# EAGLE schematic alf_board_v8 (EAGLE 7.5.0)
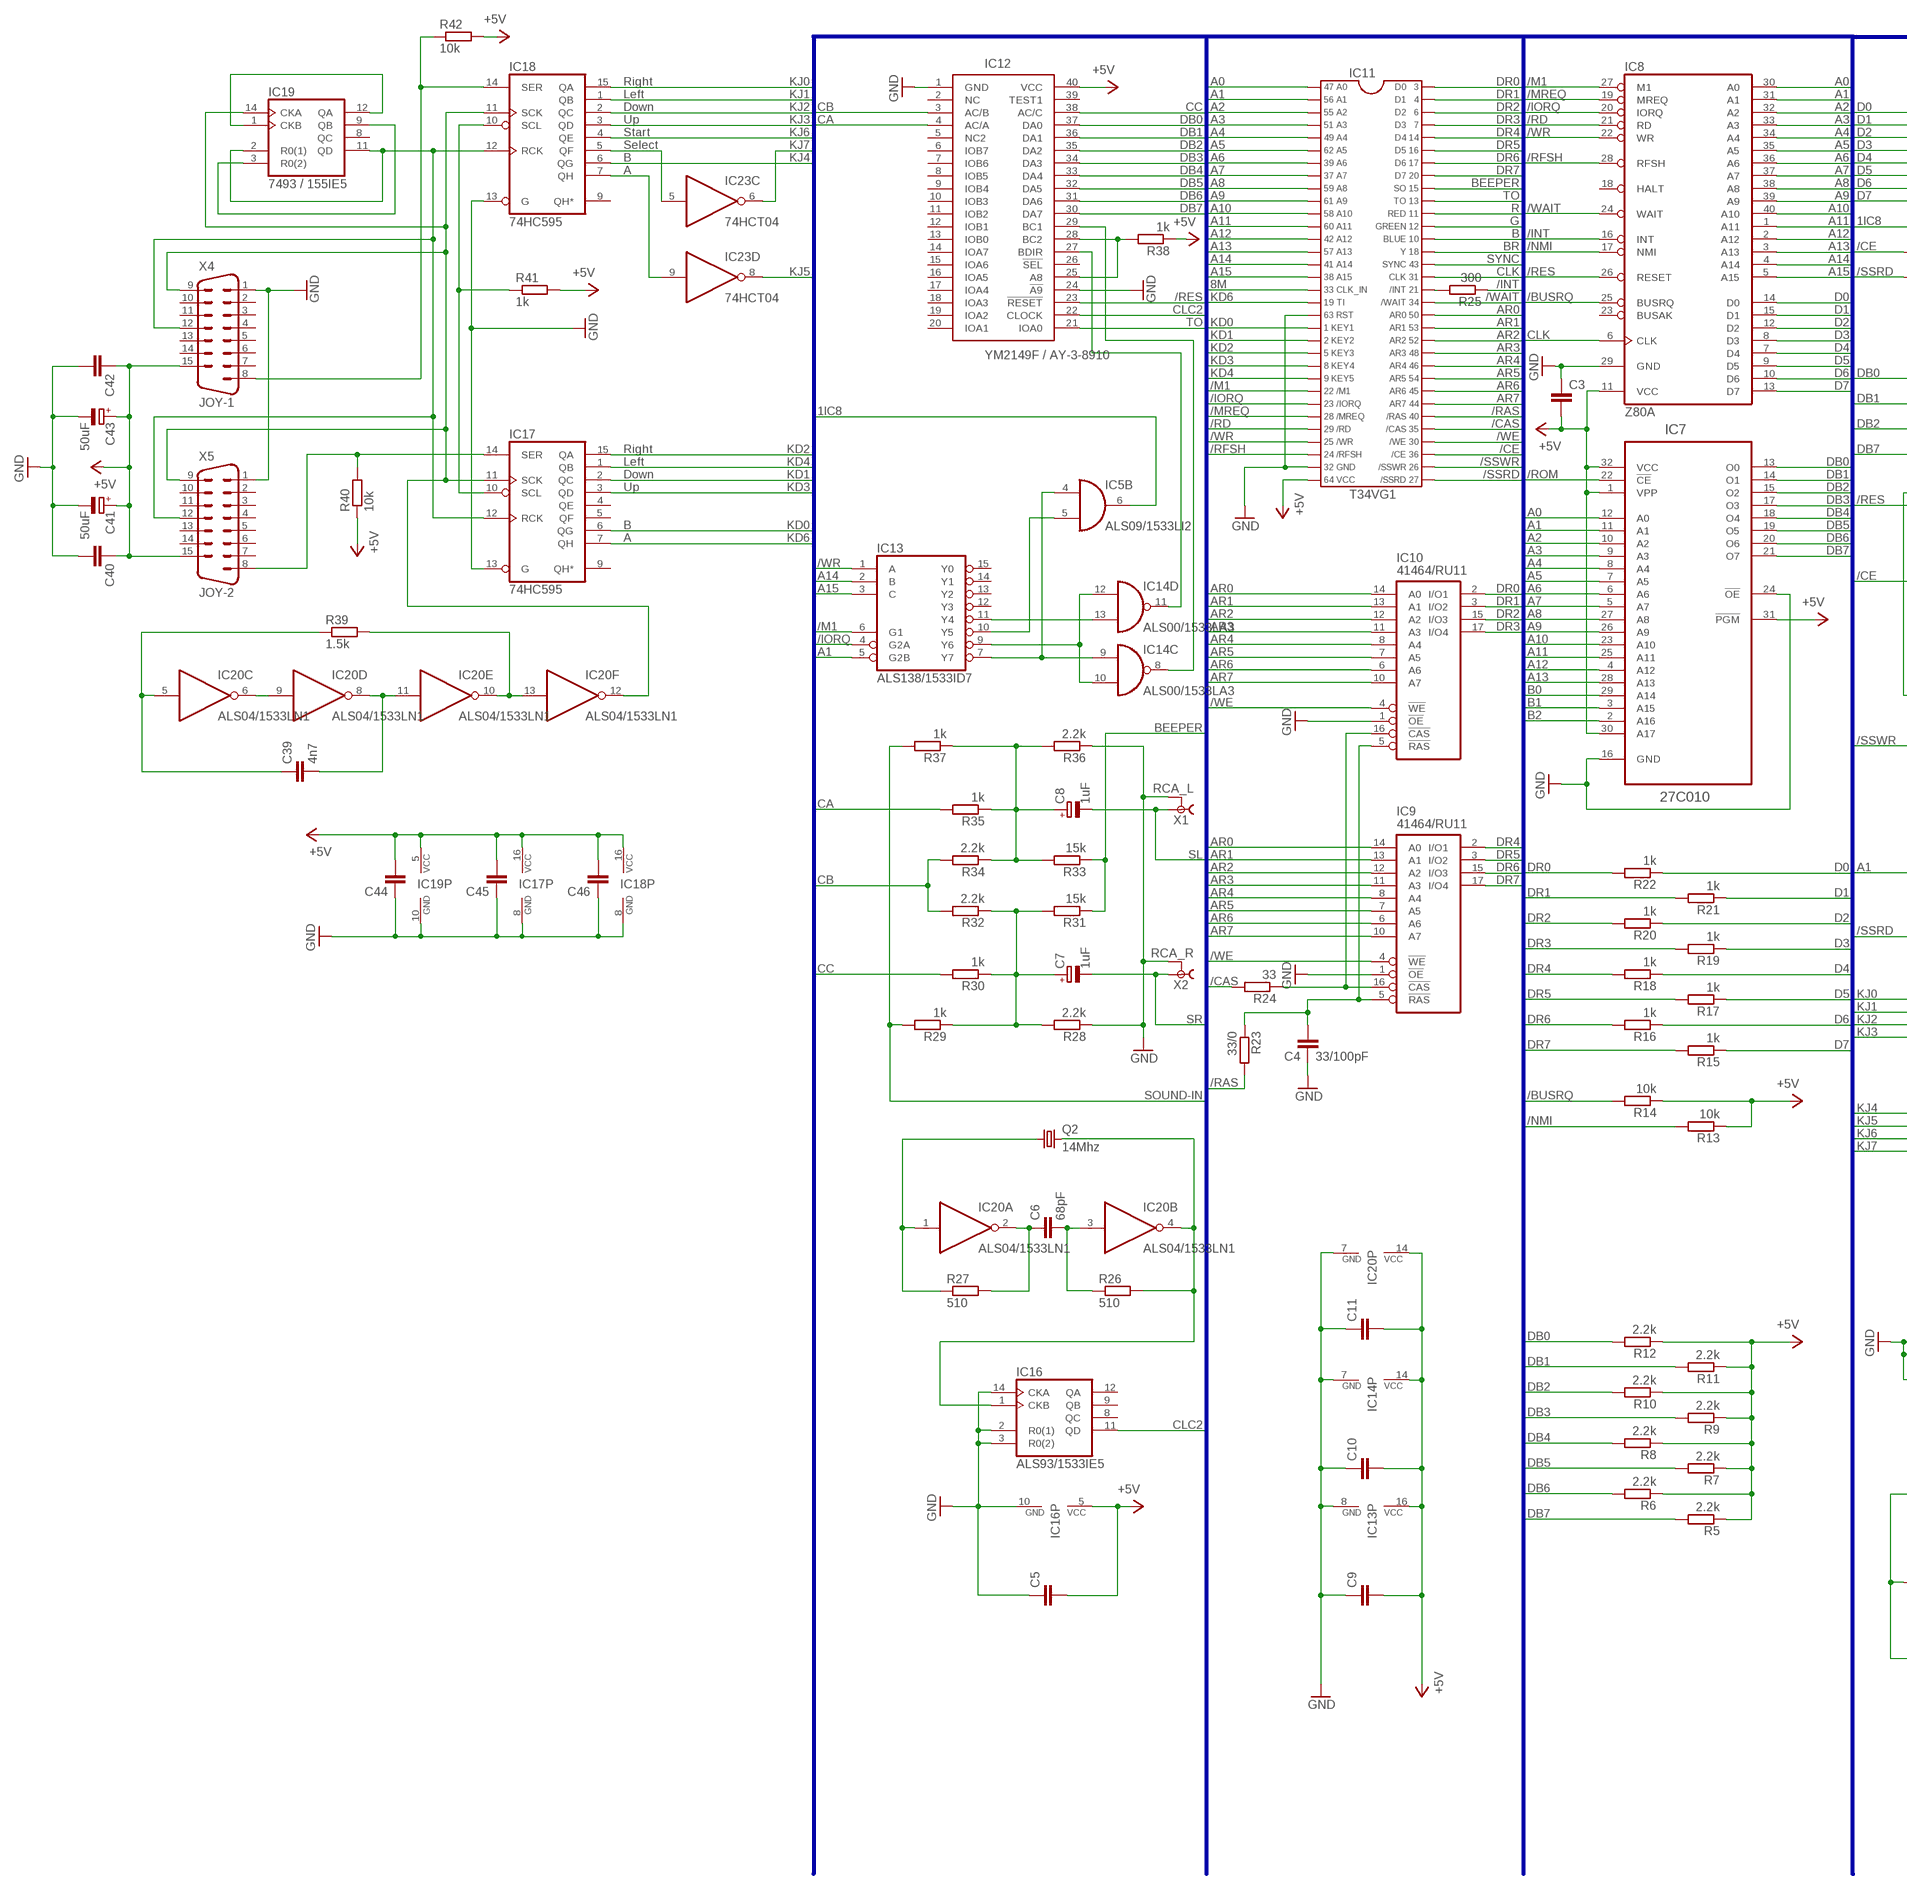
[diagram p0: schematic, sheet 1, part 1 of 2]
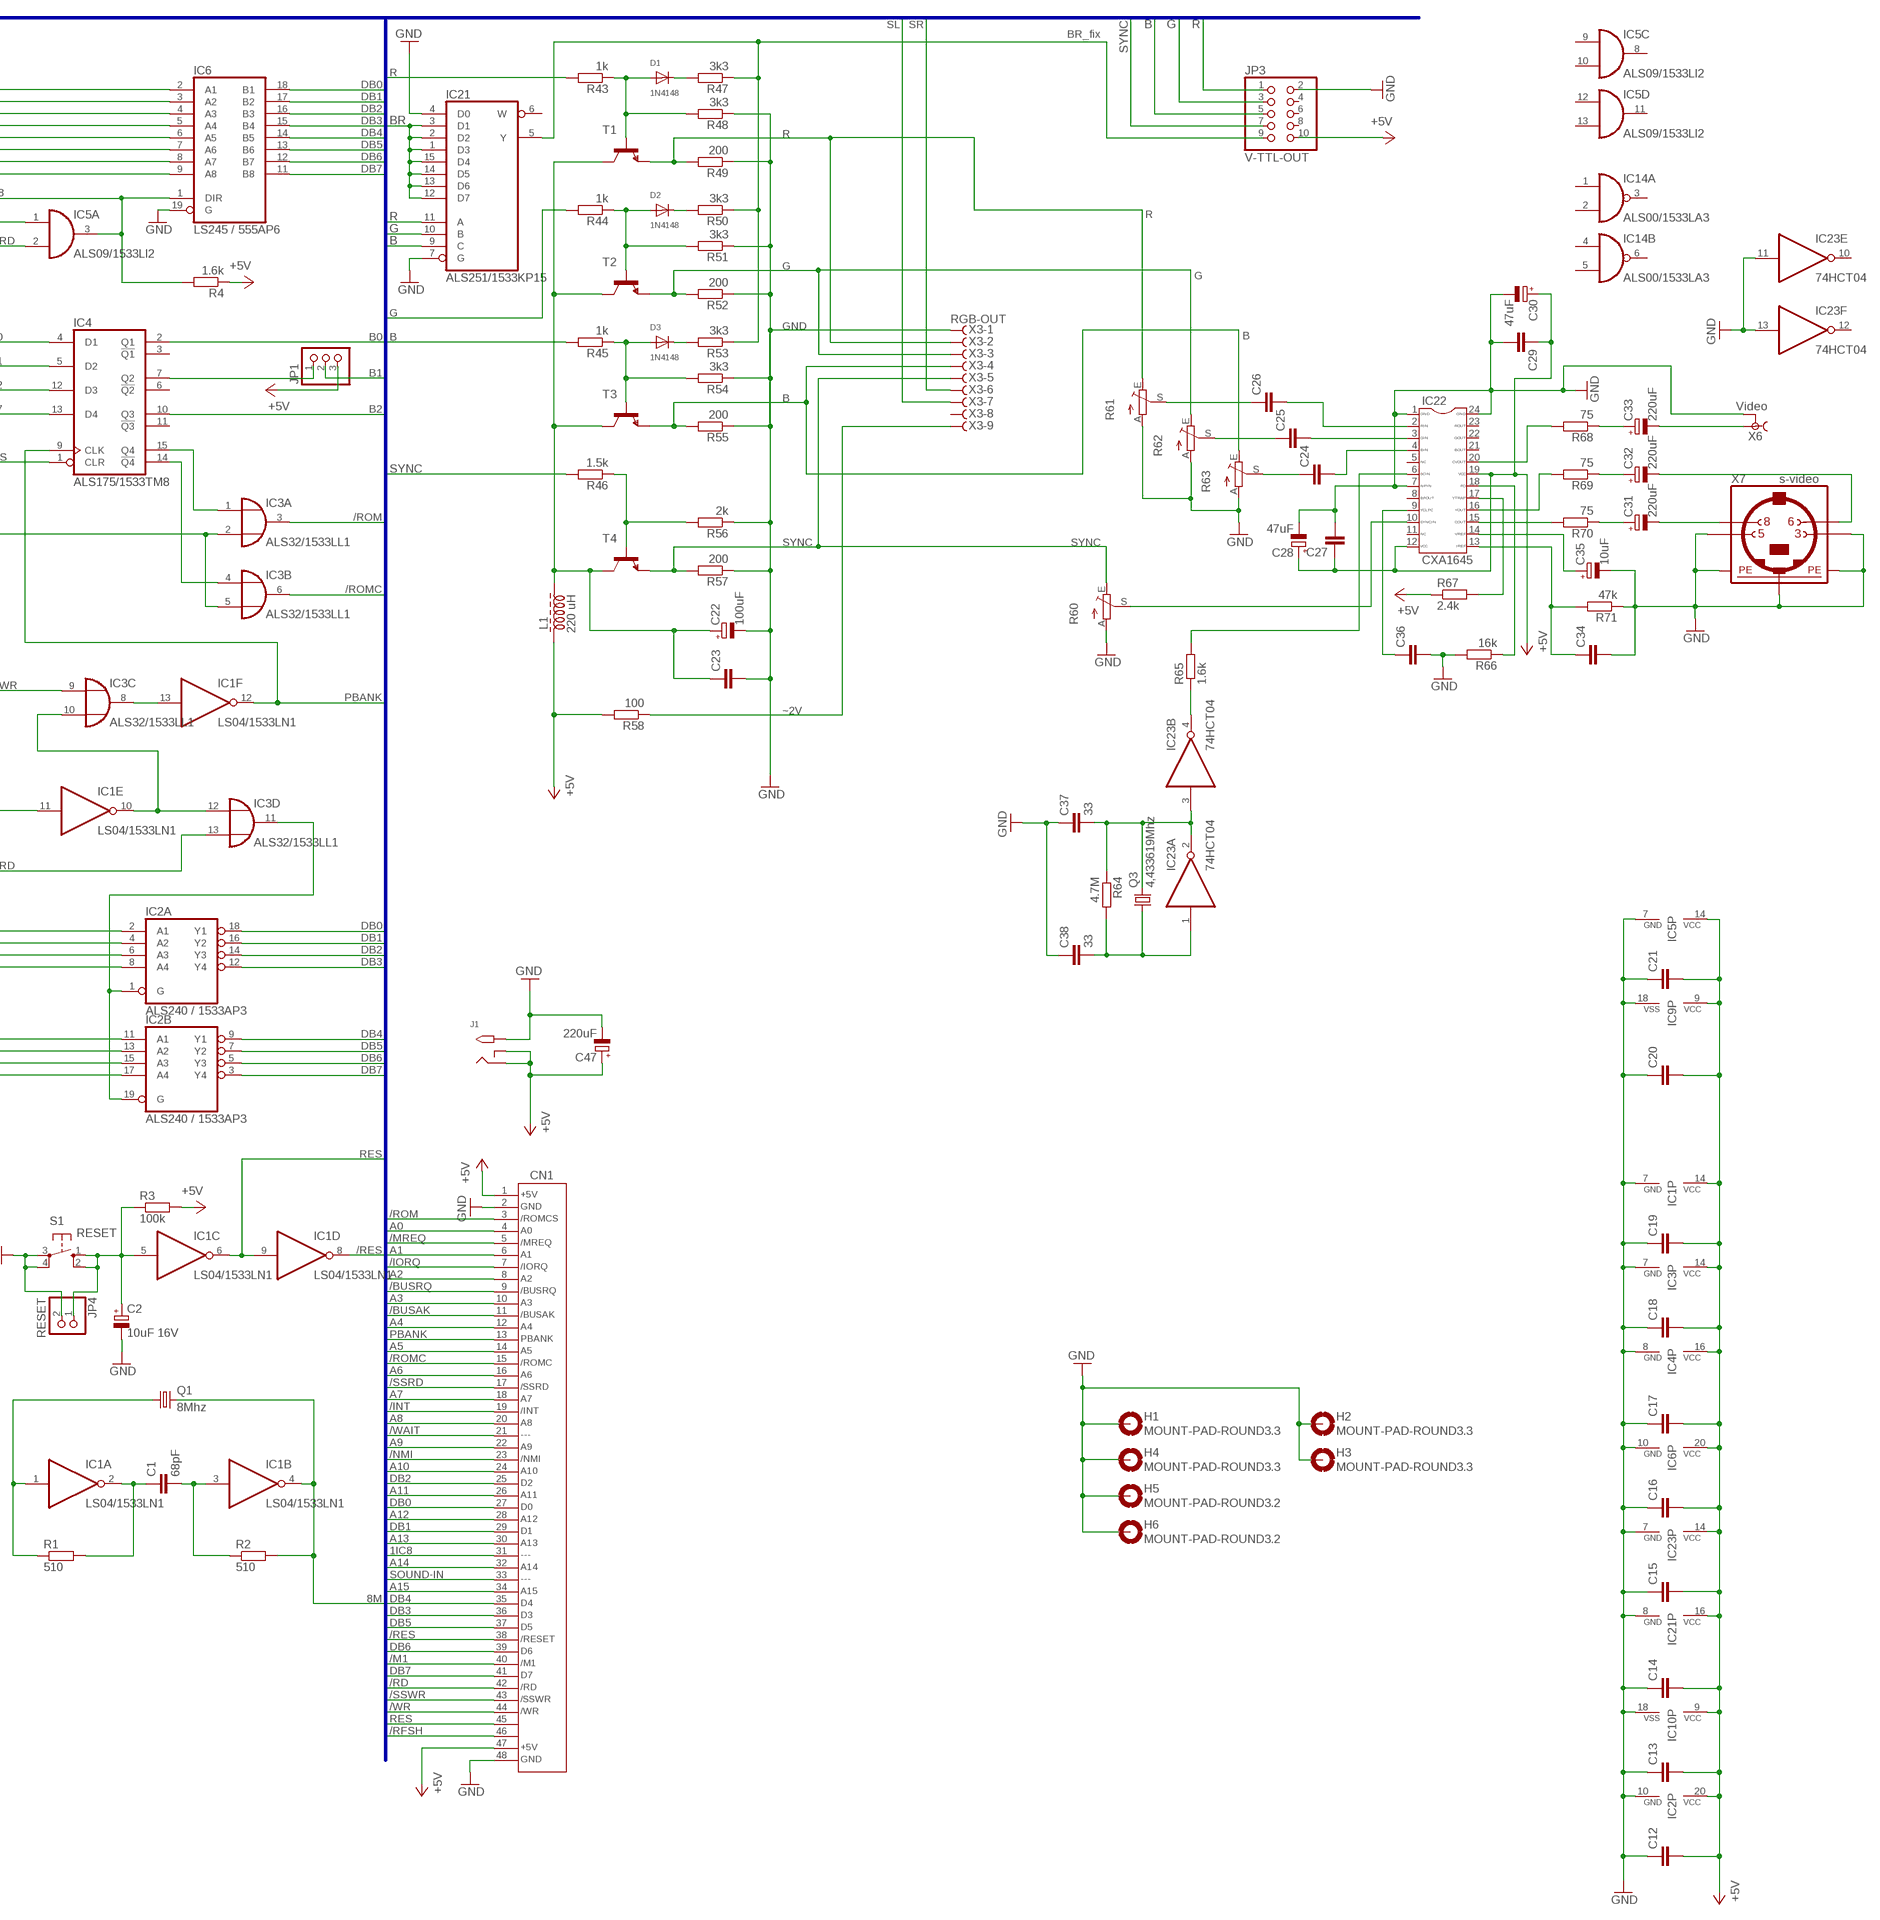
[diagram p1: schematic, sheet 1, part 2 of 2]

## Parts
C1  68pF  C-EUC0805  [C0805]
C2  10uF 16V  CPOL-EUSMCA  [SMC_A]
C3  C-EUC0805  [C0805]
C4  33/100pF  C-EUC0805  [C0805]
C5  C-EUC0805  [C0805]
C6  68pF  C-EUC0805  [C0805]
C7  1uF  CPOL-EUSMCA  [SMC_A]
C8  1uF  CPOL-EUSMCA  [SMC_A]
C9  C-EUC0805  [C0805]
C10  C-EUC0805  [C0805]
C11  C-EUC0805  [C0805]
C12  C-EUC0805  [C0805]
C13  C-EUC0805  [C0805]
C14  C-EUC0805  [C0805]
C15  C-EUC0805  [C0805]
C16  C-EUC0805  [C0805]
C17  C-EUC0805  [C0805]
C18  C-EUC0805  [C0805]
C19  C-EUC0805  [C0805]
C20  C-EUC0805  [C0805]
C21  C-EUC0805  [C0805]
C22  100uF  CPOL-EUSMCB  [SMC_B]
C23  C-EUC0805  [C0805]
C24  C-EUC0805  [C0805]
C25  C-EUC0805  [C0805]
C26  C-EUC0805  [C0805]
C27  C-EUC0805  [C0805]
C28  47uF  CPOL-EUSMCB  [SMC_B]
C29  C-EUC0805  [C0805]
C30  47uF  CPOL-EUSMCB  [SMC_B]
C31  220uF  CPOL-EUSMCD  [SMC_D]
C32  220uF  CPOL-EUSMCD  [SMC_D]
C33  220uF  CPOL-EUSMCD  [SMC_D]
C34  C-EUC0805  [C0805]
C35  10uF  CPOL-EUSMCA  [SMC_A]
C36  C-EUC0805  [C0805]
C37  33  C-EUC0805  [C0805]
C38  33  C-EUC0805  [C0805]
C39  4n7  C-EUC0805  [C0805]
C40  C-EUC0805  [C0805]
C41  50uF  CPOL-EUSMCB  [SMC_B]
C42  C-EUC0805  [C0805]
C43  50uF  CPOL-EUSMCB  [SMC_B]
C44  C-EUC0805  [C0805]
C45  C-EUC0805  [C0805]
C46  C-EUC0805  [C0805]
C47  220uF  CPOL-EUSMCD  [SMC_D]
CN1  СНП15-48  [СНП15-48]
D1  1N4148  DIODEDO-1N4148  [DO-1N4148]
D2  1N4148  DIODEDO-1N4148  [DO-1N4148]
D3  1N4148  DIODEDO-1N4148  [DO-1N4148]
H1  MOUNT-PAD-ROUND3.3  [3,3-PAD]
H2  MOUNT-PAD-ROUND3.3  [3,3-PAD]
H3  MOUNT-PAD-ROUND3.3  [3,3-PAD]
H4  MOUNT-PAD-ROUND3.3  [3,3-PAD]
H5  MOUNT-PAD-ROUND3.2  [3,2-PAD]
H6  MOUNT-PAD-ROUND3.2  [3,2-PAD]
IC1  LS04/1533LN1  74LS04N  [DIL14]
IC2  ALS240 / 1533AP3  74LS240N  [DIL20]
IC3  ALS32/1533LL1  74LS32N  [DIL14]
IC4  ALS175/1533TM8  74LS175N  [DIL16]
IC5  ALS09/1533LI2  74LS09N  [DIL14]
IC6  LS245 / 555AP6  74LS245N  [DIL20]
IC7  27C010  AT27C020-90PU  [DIP254P1524X482-32P]
IC8  Z80A  Z80CPU  [DIL40]
IC9  41464/RU11  41464  [DIL18]
IC10  41464/RU11  41464  [DIL18]
IC11  T34VG1  Т34ВГ1  [TQFP64]
IC12  YM2149F / AY-3-8910  YM2149F  [DIL40]
IC13  ALS138/1533ID7  74LS138N  [DIL16]
IC14  ALS00/1533LA3  74LS00N  [DIL14]
IC16  ALS93/1533IE5  74LS93N  [DIL14]
IC17  74HC595  74HC595N  [DIL16]
IC18  74HC595  74HC595N  [DIL16]
IC19  7493 / 155IE5  74LS93N  [DIL14]
IC20  ALS04/1533LN1  74LS04N  [DIL14]
IC21  ALS251/1533KP15  74LS251N  [DIL16]
IC22  CXA1645  [SOP24]
IC23  74HCT04  74HCT04N  [DIL14]
J1  2.1MMJACKTHM  [PJ-102A]
JP1  PINHD-1X3  [1X03]
JP3  V-TTL-OUT  PINHD-2X5  [2X05]
JP4  RESET  PINHD-1X2  [1X02]
L1  220 uH  Z27/24CW  [Z27/24]
Q1  8Mhz  CRYSTALHC49S  [HC49/S]
Q2  14Mhz  CRYSTALHC49S  [HC49/S]
Q3  4,433619Mhz  CRYSTALHC49S  [HC49/S]
R1  510  R-EU_R0805  [R0805]
R2  510  R-EU_R0805  [R0805]
R3  100k  R-EU_R0805  [R0805]
R4  1.6k  R-EU_R0805  [R0805]
R5  2.2k  R-EU_R0805  [R0805]
R6  2.2k  R-EU_R0805  [R0805]
R7  2.2k  R-EU_R0805  [R0805]
R8  2.2k  R-EU_R0805  [R0805]
R9  2.2k  R-EU_R0805  [R0805]
R10  2.2k  R-EU_R0805  [R0805]
R11  2.2k  R-EU_R0805  [R0805]
R12  2.2k  R-EU_R0805  [R0805]
R13  10k  R-EU_R0805  [R0805]
R14  10k  R-EU_R0805  [R0805]
R15  1k  R-EU_R0805  [R0805]
R16  1k  R-EU_R0805  [R0805]
R17  1k  R-EU_R0805  [R0805]
R18  1k  R-EU_R0805  [R0805]
R19  1k  R-EU_R0805  [R0805]
R20  1k  R-EU_R0805  [R0805]
R21  1k  R-EU_R0805  [R0805]
R22  1k  R-EU_R0805  [R0805]
R23  33/0  R-EU_R0805  [R0805]
R24  33  R-EU_R0805  [R0805]
R25  300  R-EU_R0805  [R0805]
R26  510  R-EU_R0805  [R0805]
R27  510  R-EU_R0805  [R0805]
R28  2.2k  R-EU_R0805  [R0805]
R29  1k  R-EU_R0805  [R0805]
R30  1k  R-EU_R0805  [R0805]
R31  15k  R-EU_R0805  [R0805]
R32  2.2k  R-EU_R0805  [R0805]
R33  15k  R-EU_R0805  [R0805]
R34  2.2k  R-EU_R0805  [R0805]
R35  1k  R-EU_R0805  [R0805]
R36  2.2k  R-EU_R0805  [R0805]
R37  1k  R-EU_R0805  [R0805]
R38  1k  R-EU_R0805  [R0805]
R39  1.5k  R-EU_R0805  [R0805]
R40  10k  R-EU_R0805  [R0805]
R41  1k  R-EU_R0805  [R0805]
R42  10k  R-EU_R0805  [R0805]
R43  1k  R-EU_R0805  [R0805]
R44  1k  R-EU_R0805  [R0805]
R45  1k  R-EU_R0805  [R0805]
R46  1.5k  R-EU_R0805  [R0805]
R47  3k3  R-EU_R0805  [R0805]
R48  3k3  R-EU_R0805  [R0805]
R49  200  R-EU_R0805  [R0805]
R50  3k3  R-EU_R0805  [R0805]
R51  3k3  R-EU_R0805  [R0805]
R52  200  R-EU_R0805  [R0805]
R53  3k3  R-EU_R0805  [R0805]
R54  3k3  R-EU_R0805  [R0805]
R55  200  R-EU_R0805  [R0805]
R56  2k  R-EU_R0805  [R0805]
R57  200  R-EU_R0805  [R0805]
R58  100  R-EU_R0805  [R0805]
R60  TRIM_EU-CA6V  [CA6V]
R61  TRIM_EU-CA6V  [CA6V]
R62  TRIM_EU-CA6V  [CA6V]
R63  TRIM_EU-CA6V  [CA6V]
R64  4.7M  R-EU_R0805  [R0805]
R65  1.6k  R-EU_R0805  [R0805]
R66  16k  R-EU_R0805  [R0805]
R67  2.4k  R-EU_R0805  [R0805]
R68  75  R-EU_R0805  [R0805]
R69  75  R-EU_R0805  [R0805]
R70  75  R-EU_R0805  [R0805]
R71  47k  R-EU_R0805  [R0805]
S1  RESET  10-XX  [B3F-10XX]
T1  BC549-NPN-TO92-CBE  [TO92-CBE]
T2  BC549-NPN-TO92-CBE  [TO92-CBE]
T3  BC549-NPN-TO92-CBE  [TO92-CBE]
T4  BC549-NPN-TO92-CBE  [TO92-CBE]
X1  RCA_L  TOBU3  [TOBU3]
X2  RCA_R  TOBU3  [TOBU3]
X3  RGB-OUT  D-SUB9-H5M09RA  [H5M09RA]
X4  JOY-1  M15HP  [M15HP]
X5  JOY-2  M15HP  [M15HP]
X6  Video  TOBU3  [TOBU3]
X7  s-video  MINI_DIN_4  [M_DIN4]

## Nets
1IC8: CN1.31 IC5.3(A:O) IC5.6(B:O) IC6.1(DIR) R4.2
8M: IC1.4(B:O) IC11.33 Q1.2 R2.2
+5V: C3.2 C5.2 C9.2 C10.2 C11.2 C12.2 C13.2 C14.2 C15.2 C16.2 C17.2 C18.2 C19.2 C20.2 C21.2 C27.1 C28.+ C29.1 C30.+ C40.1 C41.+ C42.1 C43.+ C44.2 C45.2 C46.2 C47.+ CN1.1 CN1.47 IC1.14(P:VCC) IC2.20(P:VCC) IC3.14(P:VCC) IC4.16(VCC) IC5.14(P:VCC) IC6.20(VCC) IC7.1(VPP) IC7.30(A17) IC7.31(!PGM) IC7.32(VCC) IC8.11(VCC) IC9.9(VCC) IC10.9(VCC) IC11.64 IC12.40(VCC) IC13.16(VCC) IC14.14(P:VCC) IC16.5(VCC) IC17.16(VCC) IC18.16(VCC) IC19.5(VCC) IC20.14(P:VCC) IC21.16(VCC) IC22.12 IC22.19 IC23.14(P:VCC) J1.RING J1.RING_SW JP1.3 JP3.10 L1.1 R3.2 R4.1 R5.1 R6.1 R7.1 R8.1 R9.1 R10.1 R11.1 R12.1 R13.1 R14.1 R38.1 R40.1 R41.2 R42.2 R58.2 R67.1 X4.15 X5.15
/BUSAK: CN1.11
/BUSRQ: CN1.9 IC8.25(BUSRQ) R14.2
/CAS: IC11.35 R24.2
/CE: IC3.2(A:I1) IC3.5(B:I1) IC5.1(A:I0) IC11.36
/INT: CN1.19 IC8.16(INT) R25.1
/IORQ: CN1.7 IC8.20(IORQ) IC11.23 IC13.4(G2A)
/M1: CN1.40 IC8.27(M1) IC11.22 IC13.6(G1)
/MREQ: CN1.5 IC8.19(MREQ) IC11.28
/NMI: CN1.23 IC8.17(NMI) R13.2
/RAS: IC11.40 R23.2
/RD: CN1.42 IC8.21(RD) IC11.29
/RES: CN1.38 IC1.8(D:O) IC4.1(CLR) IC8.26(RESET) IC12.23(!RESET)
/RFSH: CN1.46 IC8.28(RFSH) IC11.24
/ROM: CN1.3 IC3.3(A:O) IC7.22(!CE)
/ROMC: CN1.15 IC3.6(B:O)
/SSRD: CN1.17 IC3.13(D:I1) IC5.2(A:I1) IC11.27
/SSWR: CN1.43 IC3.9(C:I0) IC11.26
/WAIT: CN1.21 IC8.24(WAIT) IC11.34
/WE: IC9.4(!WE) IC10.4(!WE) IC11.30
/WR: CN1.44 IC8.22(WR) IC11.25 IC13.1(A)
A0: CN1.4 IC7.12(A0) IC8.30(A0) IC11.47
A1: CN1.6 IC1.11(E:I) IC7.11(A1) IC8.31(A1) IC11.56 IC13.5(G2B)
A2: CN1.8 IC7.10(A2) IC8.32(A2) IC11.55
A3: CN1.10 IC7.9(A3) IC8.33(A3) IC11.51
A4: CN1.12 IC7.8(A4) IC8.34(A4) IC11.49
A5: CN1.14 IC7.7(A5) IC8.35(A5) IC11.62
A6: CN1.16 IC7.6(A6) IC8.36(A6) IC11.39
A7: CN1.18 IC7.5(A7) IC8.37(A7) IC11.37
A8: CN1.20 IC7.27(A8) IC8.38(A8) IC11.59
A9: CN1.22 IC7.26(A9) IC8.39(A9) IC11.61
A10: CN1.24 IC7.23(A10) IC8.40(A10) IC11.58
A11: CN1.26 IC7.25(A11) IC8.1(A11) IC11.60
A12: CN1.28 IC7.4(A12) IC8.2(A12) IC11.42
A13: CN1.30 IC7.28(A13) IC8.3(A13) IC11.57
A14: CN1.32 IC8.4(A14) IC11.41 IC13.2(B)
A15: CN1.34 IC8.5(A15) IC11.38 IC13.3(C)
AR0: IC9.14(A0) IC10.14(A0) IC11.50
AR1: IC9.13(A1) IC10.13(A1) IC11.53
AR2: IC9.12(A2) IC10.12(A2) IC11.52
AR3: IC9.11(A3) IC10.11(A3) IC11.48
AR4: IC9.8(A4) IC10.8(A4) IC11.46
AR5: IC9.7(A5) IC10.7(A5) IC11.54
AR6: IC9.6(A6) IC10.6(A6) IC11.45
AR7: IC9.10(A7) IC10.10(A7) IC11.44
B: IC11.10 IC21.9(C) JP3.5 R45.2
B0: IC4.2(Q1) IC7.29(A14)
B1: IC7.3(A15) JP1.2
B2: IC4.10(Q3) IC7.2(A16)
BEEPER: IC11.15 R31.1 R33.1
BR: IC11.18 IC21.1(D3) IC21.2(D2) IC21.3(D1) IC21.12(D7) IC21.13(D6) IC21.14(D5) IC21.15(D4)
CA: IC12.4(AC/A) R35.2
CB: IC12.3(AC/B) R32.2 R34.2
CC: IC12.38(AC/C) R30.2
CLC2: IC12.22(CLOCK) IC16.11(QD)
CLK: IC8.6(CLK) IC11.31
D0: IC6.2(A1) IC8.14(D0) R22.1
D1: IC6.3(A2) IC8.15(D1) R21.1
D2: IC6.4(A3) IC8.12(D2) R20.1
D3: IC6.5(A4) IC8.8(D3) R19.1
D4: IC6.6(A5) IC8.7(D4) R18.1
D5: IC6.7(A6) IC8.9(D5) R17.1
D6: IC6.8(A7) IC8.10(D6) R16.1
D7: IC6.9(A8) IC8.13(D7) R15.1
DB0: CN1.27 IC2.18(A:Y1) IC4.4(D1) IC6.18(B1) IC7.13(O0) IC12.37(DA0) R12.2
DB1: CN1.29 IC2.16(A:Y2) IC4.5(D2) IC6.17(B2) IC7.14(O1) IC12.36(DA1) R11.2
DB2: CN1.25 IC2.14(A:Y3) IC4.12(D3) IC6.16(B3) IC7.15(O2) IC12.35(DA2) R10.2
DB3: CN1.36 IC2.12(A:Y4) IC6.15(B4) IC7.17(O3) IC12.34(DA3) R9.2
DB4: CN1.35 IC2.9(B:Y1) IC6.14(B5) IC7.18(O4) IC12.33(DA4) R8.2
DB5: CN1.37 IC2.7(B:Y2) IC6.13(B6) IC7.19(O5) IC12.32(DA5) R7.2
DB6: CN1.39 IC2.5(B:Y3) IC6.12(B7) IC7.20(O6) IC12.31(DA6) R6.2
DB7: CN1.41 IC2.3(B:Y4) IC4.13(D4) IC6.11(B8) IC7.21(O7) IC12.30(DA7) R5.2
DR0: IC10.2(I/O1) IC11.3 R22.2
DR1: IC10.3(I/O2) IC11.4 R21.2
DR2: IC10.15(I/O3) IC11.6 R20.2
DR3: IC10.17(I/O4) IC11.7 R19.2
DR4: IC9.2(I/O1) IC11.14 R18.2
DR5: IC9.3(I/O2) IC11.16 R17.2
DR6: IC9.15(I/O3) IC11.17 R16.2
DR7: IC9.17(I/O4) IC11.20 R15.2
G: IC11.12 IC21.10(B) JP3.3 R44.2
GND: C2.- C3.1 C4.1 C5.1 C9.1 C10.1 C11.1 C12.1 C13.1 C14.1 C15.1 C16.1 C17.1 C18.1 C19.1 C20.1 C21.1 C22.- C23.2 C27.2 C28.- C29.2 C30.- C34.2 C35.- C36.2 C37.1 C38.1 C40.2 C41.- C42.2 C43.- C44.1 C45.1 C46.1 C47.- CN1.2 CN1.48 H1.B3,3(MOUNT) H2.B3,3(MOUNT) H3.B3,3(MOUNT) H4.B3,3(MOUNT) H5.B3,2(MOUNT) H6.B3,2(MOUNT) IC1.7(P:GND) IC2.10(P:GND) IC3.7(P:GND) IC4.8(GND) IC5.7(P:GND) IC6.10(GND) IC6.19(G) IC7.16(GND) IC7.24(!OE) IC8.29(GND) IC9.1(!OE) IC9.18(VSS) IC10.1(!OE) IC10.18(VSS) IC11.32 IC11.63 IC12.1(GND) IC12.24(!A9) IC13.8(GND) IC14.7(P:GND) IC16.2(R0(1)) IC16.3(R0(2)) IC16.10(GND) IC16.14(CKA) IC17.8(GND) IC17.13(G) IC18.8(GND) IC18.13(G) IC19.10(GND) IC20.7(P:GND) IC21.4(D0) IC21.7(G) IC21.8(GND) IC22.1 IC22.7 IC22.24 IC23.7(P:GND) IC23.11(E:I) IC23.13(F:I) J1.TIP JP3.2 JP4.2 R28.1 R36.1 R48.1 R49.1 R51.1 R52.1 R54.1 R55.1 R56.1 R57.1 R60.A R61.A R62.A R63.A R66.2 R71.1 S1.3(P) S1.4(P1) X1.2 X1.2@1 X1.2@2 X2.2 X2.2@1 X2.2@2 X3.1 X4.1 X5.1 X6.2 X6.2@1 X6.2@2 X7.3 X7.5 X7.SH1(PE1) X7.SH2(PE2) X7.SH3(PE3)
KD0: IC11.1 IC17.6(QG)
KD1: IC11.2 IC17.2(QC)
KD2: IC11.5 IC17.15(QA)
KD3: IC11.8 IC17.3(QD)
KD4: IC11.9 IC17.1(QB)
KD6: IC11.19 IC17.7(QH)
KJ0: IC2.2(A:A1) IC18.15(QA)
KJ1: IC2.4(A:A2) IC18.1(QB)
KJ2: IC2.6(A:A3) IC18.2(QC)
KJ3: IC2.8(A:A4) IC18.3(QD)
KJ4: IC2.11(B:A1) IC18.6(QG)
KJ5: IC2.13(B:A2) IC23.8(D:O)
KJ6: IC2.15(B:A3) IC18.4(QE)
KJ7: IC2.17(B:A4) IC23.6(C:O)
N$1: IC23.4(B:O) R65.1
N$2: C1.1 IC1.2(A:O) R1.2
N$3: C1.2 IC1.3(B:I) R2.1
N$4: IC1.1(A:I) Q1.1 R1.1
N$5: IC18.5(QF) IC23.5(C:I)
N$6: IC18.7(QH) IC23.9(D:I)
N$7: IC1.13(F:I) IC3.8(C:O)
N$8: C2.+ IC1.5(C:I) JP4.1 R3.1 S1.1(S) S1.2(S1)
N$9: IC4.7(Q2) JP1.1
N$10: IC1.10(E:O) IC3.10(C:I1) IC3.12(D:I0)
N$11: IC3.4(B:I0) IC4.14(!Q4)
N$12: IC2.1(A:G) IC2.19(B:G) IC3.11(D:O)
N$13: IC3.1(A:I0) IC4.15(Q4)
N$14: IC17.12(RCK) IC18.12(RCK) IC19.2(R0(1)) IC19.11(QD) X4.12 X5.12
N$15: IC11.21 R25.2
N$16: IC12.25(A8) IC12.28(BC2) R38.2
N$17: D1.A R43.1 R48.2 T1.B
N$18: D1.C R47.2
N$19: R49.2 R61.E T1.E X3.2
N$21: D2.A R44.1 R51.2 T2.B
N$22: D2.C R50.2
N$23: R52.2 R62.E T2.E X3.3
N$24: IC22.17 R67.2
N$25: IC12.27(BDIR) IC14.11(D:O)
N$26: IC5.4(B:I0) IC13.7(Y7) IC14.9(C:I0)
N$27: IC13.11(Y4) IC14.13(D:I1)
N$28: IC5.5(B:I1) IC13.10(Y5)
N$29: IC13.9(Y6) IC14.10(C:I1) IC14.12(D:I0)
N$30: IC17.10(SCL) IC18.10(SCL) R41.1
N$31: IC12.29(BC1) IC14.8(C:O)
N$32: C8.+ R33.2 R34.1 R35.1 R36.2 R37.1
N$33: C7.+ R28.2 R29.1 R30.1 R31.2 R32.1
N$34: D3.A R45.1 R54.2 T3.B
N$35: IC17.11(SCK) IC18.11(SCK) IC19.14(CKA) IC20.12(F:O) X4.9 X5.9
N$36: C39.1 IC20.5(C:I) R39.1
N$37: IC16.1(CKB) IC20.4(B:O) Q2.2 R26.2
N$38: IC20.1(A:I) Q2.1 R27.1
N$39: C6.1 IC20.2(A:O) R27.2
N$40: C6.2 IC20.3(B:I) R26.1
N$41: D3.C R53.2
N$42: R55.2 R63.E T3.E X3.4
N$43: R57.2 R60.E T4.E X3.5
N$44: C22.+ C23.1 L1.2 T1.C T2.C T3.C T4.C
N$45: R58.1 X3.9
N$46: IC17.14(SER) R40.2 X5.8
N$47: IC19.3(R0(2)) IC19.9(QB)
N$48: IC18.14(SER) R42.1 X4.8
N$49: IC19.1(CKB) IC19.12(QA)
N$50: C39.2 IC20.8(D:O) IC20.11(E:I)
N$51: IC20.10(E:O) IC20.13(F:I) R39.2
N$52: C26.1 R61.S
N$53: IC20.6(C:O) IC20.9(D:I)
N$54: C25.1 R62.S
N$55: C24.1 R63.S
N$56: C25.2 IC22.3
N$57: C26.2 IC22.2
N$58: C24.2 IC22.4
N$59: C38.2 IC23.1(A:I) Q3.1 R64.2
N$60: C37.2 IC23.2(A:O) IC23.3(B:I) Q3.2 R64.1
N$61: IC22.10 R60.S
N$62: IC21.5(Y) JP3.9 R47.1 R50.1 R53.1
N$63: IC22.6 R65.2
N$64: IC22.20 R68.2
N$65: C36.1 IC22.9
N$66: IC22.18 R66.1
N$67: IC22.16 R69.2
N$68: IC22.15 R70.2
N$69: C33.+ R68.1
N$70: C32.+ R69.1
N$71: C31.+ R70.1
N$72: C35.+ IC22.14
N$73: C34.1 IC22.13 R71.2
N$75: C33.- X6.1
N$76: IC9.16(!CAS) IC10.16(!CAS) R24.1
N$77: C4.2 IC9.5(!RAS) IC10.5(!RAS) R23.1
N$78: C32.- X7.6
N$79: C31.- X7.8
N$126: R46.1 R56.2 T4.B
PBANK: CN1.13 IC1.12(F:O) IC4.9(CLK)
R: IC11.11 IC21.11(A) JP3.1 R43.2
RES: CN1.45 IC1.6(C:O) IC1.9(D:I)
SL: C8.- X1.1 X3.7
SOUND-IN: CN1.33 R29.2 R37.2
SR: C7.- X2.1 X3.6
SYNC: IC11.43 JP3.7 R46.2
TO: IC11.13 IC12.21(IOA0)
Unconnected: IC4.3(!Q1) IC4.6(!Q2) IC4.11(!Q3) IC5.8(C:O) IC5.9(C:I0) IC5.10(C:I1) IC5.11(D:O) IC5.12(D:I0) IC5.13(D:I1) IC8.18(HALT) IC8.23(BUSAK) IC12.2(NC) IC12.5(NC2) IC12.6(IOB7) IC12.7(IOB6) IC12.8(IOB5) IC12.9(IOB4) IC12.10(IOB3) IC12.11(IOB2) IC12.12(IOB1) IC12.13(IOB0) IC12.14(IOA7) IC12.15(IOA6) IC12.16(IOA5) IC12.17(IOA4) IC12.18(IOA3) IC12.19(IOA2) IC12.20(IOA1) IC12.26(!SEL) IC12.39(TEST1) IC13.12(Y3) IC13.13(Y2) IC13.14(Y1) IC13.15(Y0) IC14.1(A:I0) IC14.2(A:I1) IC14.3(A:O) IC14.4(B:I0) IC14.5(B:I1) IC14.6(B:O) IC16.8(QC) IC16.9(QB) IC16.12(QA) IC17.4(QE) IC17.5(QF) IC17.9(QH*) IC18.9(QH*) IC19.8(QC) IC21.6(W) IC22.5 IC22.8 IC22.11 IC22.21 IC22.22 IC22.23 IC23.10(E:O) IC23.12(F:O) JP3.4 JP3.6 JP3.8 X3.8 X4.2 X4.3 X4.4 X4.5 X4.6 X4.7 X4.10 X4.11 X4.13 X4.14 X5.2 X5.3 X5.4 X5.5 X5.6 X5.7 X5.10 X5.11 X5.13 X5.14

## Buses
A[0..15],AR[0..7],D[0..7],DB[0..7],DR[0..7],KD[0..6],KJ[0..7],B[0..2],/ROM,/MREQ,/IORQ,/BUSRQ,/BUSAK,PBANK,/ROMC,/SSRD,/INT,/NMI,/RES,RES,/M1,/SSRD,/RD,/SSWR,/WR,/RFSH,/RAS,/CAS,/WE,/M1,/WAIT,/CE,8M,CLK,CLC2,SYNC,BR,R,G,B,CA,CB,CC,BEEPER,SR,SL,1IC8,SOUND-IN,TO

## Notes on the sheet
- BR_fix
- Right
- Left
- Down
- Up
- Start
- Select
- B | R
- A
- R
- G
- G
- GND
- B
- B
- Right
- Left
- Down
- Up
- B
- A
- SYNC | SYNC
- ~2V

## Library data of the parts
C1 C3-C6 C9-C21 C23-C27 C29 C34 C36-C40 C42 C44-C46 = rcl:C-EU: CAPACITOR, European symbol; OC_FARNELL: unknown
C2 = rcl:CPOL-EU: POLARIZED CAPACITOR, European symbol; MF: MULTICOMP; MPN: MCNP35V106M5X11; OC_FARNELL: 1236669
C7 C8 C22 C28 C30-C33 C35 C41 C43 C47 = rcl:CPOL-EU: POLARIZED CAPACITOR, European symbol; OC_FARNELL: unknown
CN1 = alf_cartridge_slot:СНП15-48; OC_FARNELL: unknown
D1-D3 = adafruit:DIODE: Diode; OC_FARNELL: unknown
H1-H6 = holes:MOUNT-PAD-ROUND: MOUNTING PAD, round
IC1 IC20 = 74xx-eu:74*04: Hex INVERTER; OC_FARNELL: unknown
IC2 = 74xx-eu:74*240: Octal BUFFER and LINE DRIVER, 3-state; OC_FARNELL: unknown
IC3 = 74xx-eu:74*32: Quad 2-input OR gate; OC_FARNELL: unknown
IC4 = 74xx-eu:74*175: Qadruple D type FLIP FLOP, clear; OC_FARNELL: unknown
IC5 = 74xx-eu:74*09: Quad 2-input AND gate, open collector; OC_FARNELL: unknown
IC6 = 74xx-eu:74*245: Octal BUS TRANSCEIVER, 3-state; OC_FARNELL: unknown
IC7 = AT27C020:AT27C020-90PU: ONE TIME PROGRAMMABLE (OTP) EPROM IC,2Mb (256K x 8),PDIP-32; MF: ATMEL; MPN: AT27C020-90PU; OC_FARNELL: 1095777; OC_NEWARK: 68T4266; PACKAGE: PDIP-32; SUPPLIER: ATMEL
IC8 = zilog:Z80CPU: Z80 FAMILY DEVICE; OC_FARNELL: unknown
IC9 IC10 = memories:41464: DRAM 64K x 4 bits; OC_FARNELL: unknown
IC11 = Т43ВГ1:Т34ВГ1; OC_FARNELL: unknown
IC12 = ym2149f:YM2149F; OC_FARNELL: unknown
IC13 = 74xx-eu:74*138: 3-line to 8-line DECODER/DEMULTIPLEXER; OC_FARNELL: unknown
IC14 = 74xx-eu:74*00: Quad 2-input NAND gate; OC_FARNELL: unknown
IC16 IC19 = 74xx-eu:74*93: Decade, divide by twelve and binary COUNTER; OC_FARNELL: unknown
IC17 IC18 = 74xx-eu:74*595: 8-bit SHIFT REGISTER, output latch; OC_FARNELL: unknown
IC21 = 74xx-eu:74*251: 1 of 8 data SELECTOR/MULTIPLEXER, 3-state; OC_FARNELL: unknown
IC22 = CXA1645M:CXA1645; OC_FARNELL: unknown
IC23 = 74xx-eu:74*04: Hex INVERTER
J1 = adafruit:2.1MMJACK: 2.1mm x 5.5mm THM DC jack with internal switch. Digikey part #PJ-102A, 4UCON part #05537 2.1mm x 5.5mm SMT DC jack with internal switch. Digikey part #PJ-002A-SMT, 4UCON part #03267 By microbuilder.eu & adafruit.com
JP1 = pinhead:PINHD-1X3: PIN HEADER; OC_FARNELL: unknown
JP3 = pinhead:PINHD-2X5: PIN HEADER; OC_FARNELL: unknown
JP4 = pinhead:PINHD-1X2: PIN HEADER
L1 = inductor-neosid:Z?CW: CHOKE; OC_FARNELL: unknown; OC_NEWARK: unknown
Q1-Q3 = crystal:CRYSTAL: CRYSTAL; MF: MULTICOMP; MPN: HC49SM-3.6864-30-50-60-16-ATF; OC_FARNELL: 1667008; OC_NEWARK: unknown
R1-R58 R64-R71 = rcl:R-EU_: RESISTOR, European symbol; OC_FARNELL: unknown
R60-R63 = pot:TRIM_EU-: POTENTIOMETER; OC_FARNELL: unknown
S1 = switch-omron:10-XX: OMRON SWITCH; MF: OMRON ELECTRONIC COMPONENTS; MPN: B3F-1000; OC_FARNELL: 176432; OC_NEWARK: 36M3542
T1-T4 = transistor:*-NPN-: NPN Transistror BF959 corrected 2008.03.06; OC_FARNELL: unknown
X1 X2 X6 = con-hirschmann:TOBU3: Female Cinch CONNECTOR ( RCA Jack ); MF: HIRSCHMANN; MPN: TOBU 3; OC_FARNELL: 592791; OC_NEWARK: 06WX5914
X3 = con-thomas-betts:D-SUB9-: D-Subminiatur Connector Source: Electronioc Interconnects European Edition 1998; OC_FARNELL: unknown; OC_NEWARK: unknown
X4 X5 = con-subd:M15: SUB-D; OC_FARNELL: unknown; OC_NEWARK: unknown
X7 = mini_din:MINI_DIN_4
